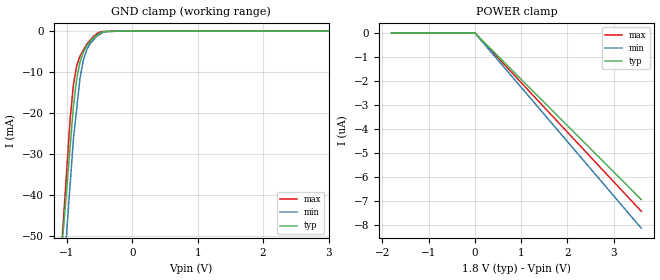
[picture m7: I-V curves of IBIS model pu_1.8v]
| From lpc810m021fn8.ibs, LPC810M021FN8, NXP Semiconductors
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[Model] pu_1.8v
Model_type Input
Vinl = 540.000mV
Vinh = 1.26000V
C_comp 909.000fF 904.000fF 914.000fF
| variable typ   min   max
[Voltage Range] 1.80000V 1.65000V 1.95000V
[POWER Clamp Reference] 1.80000V 1.65000V 1.95000V
[GND Clamp Reference] 0.00000V 0.00000V 0.00000V
[Temperature Range]   25   85   -40
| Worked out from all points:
|   GND clamp passes 1 mA (typ) near -0.54 V on its own axis
[GND Clamp]
-1.8V     -194.6mA   -224.9mA   -224.6mA
-950mV    -28.04mA   -37.26mA   -21.27mA
-900mV    -18.25mA   -26.22mA   -13mA
-850mV    -11.68mA   -18.85mA   -8.425mA
-800mV    -7.541mA   -11.48mA   -6.076mA
-750mV    -5.144mA   -7.199mA   -4.681mA
-700mV    -3.664mA   -4.647mA   -3.287mA
-650mV    -2.706mA   -3.216mA   -2.35mA
-550mV    -1.121mA   -1.325mA   -717.3uA
-400mV    -147.2uA   -119uA     -68.5uA
-200mV    -21.15uA   -16.21uA   -21.06uA
3.6V      0A         0A         0A
[POWER Clamp]
-1.8V     0A         0A         0A
0V        0A         0A         0A
3.6V      -6.941uA   -8.131uA   -7.427uA
